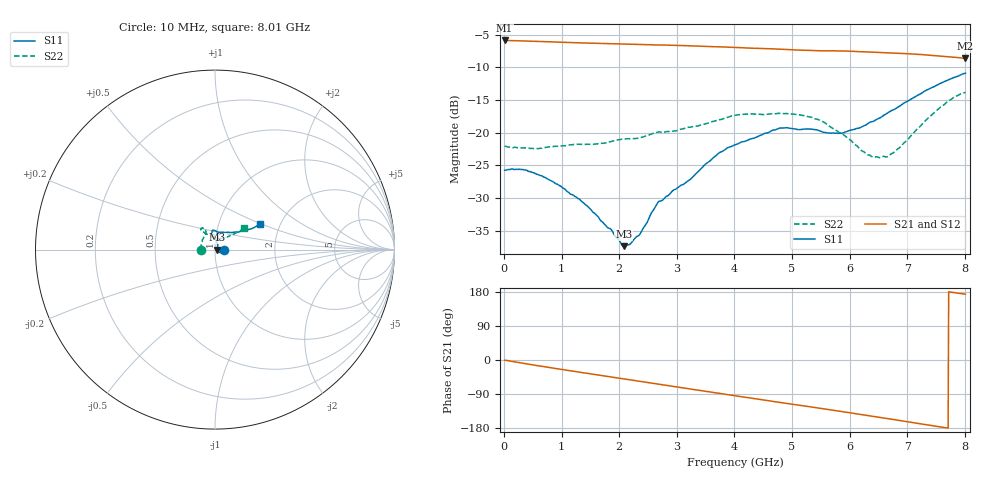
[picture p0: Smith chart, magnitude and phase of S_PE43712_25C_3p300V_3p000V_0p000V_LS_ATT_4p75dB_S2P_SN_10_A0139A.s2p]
! DEVICE ID: PE43712
! File Path: z:\PE43713\PE43713_CHAR_NOM_04292014\AMB\3p300\LS_ATT_4p75dB\PE43713_AMB_3p300V_3p000V_0p000V_LS_ATT_4p75dB_S2P_SN_10_A0139A.s2p
! Serial: 10
! Lot: A0139A
! Temp: 25C
! VDD: 3.300
! VSS: 0.000
! Control_Hi: 3.000
! Control_Lo: 0.000
! Attenuation Step: 4.75dB
! Port 1: RF1
! Port 2: RF2
! ThroughPath:1-2
! IDD: 0.0001469786
! ISS: -4.98e-008
#  Hz  S  RI  R  50
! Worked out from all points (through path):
!   801 points, 10 MHz to 8.01 GHz, reference 50 ohm
!   highest |S21| = -5.86 dB at 10 MHz (marker M1); lowest = -8.6 dB at 8.01 GHz (marker M2)
!   group delay of S21, straight-line fit = 64 ps
!   lowest |S11| = -37.4 dB at 2.08 GHz (marker M3), VSWR 1.03, Z = 51.4 + j0.00512 ohm
!   |S11| at or under -10 dB: start of sweep to end of sweep
!   |S22| runs from -23.8 to -13.8 dB; largest |S21 - S12| = 0.0015
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1e7  0.0517 -0.000115  0.5091 -0.00275  0.509 -0.00281  -0.079 0.000407
3.4e8  0.0512 -0.01  0.4982 -0.078  0.498 -0.0768  -0.0763 0.00628
6.3e8  0.0446 -0.0151  0.4803 -0.1383  0.4803 -0.1383  -0.0751 0.0123
9.6e8  0.0355 -0.0172  0.4512 -0.2009  0.4513 -0.2009  -0.0766 0.02
1.35e9  0.0255 -0.0154  0.4088 -0.2657  0.4088 -0.2658  -0.0759 0.03
1.86e9  0.0175 -0.005  0.3417 -0.3386  0.3417 -0.3385  -0.0708 0.0483
2.08e9  0.0136 4.98e-05  0.3087 -0.3656  0.3088 -0.3655  -0.0702 0.0556
2.18e9  0.0136 0.00303  0.2931 -0.3769  0.2932 -0.3767  -0.0682 0.0589
2.36e9  0.0133 0.0103  0.2632 -0.3954  0.2633 -0.3953  -0.0627 0.0668
2.68e9  0.0157 0.0252  0.2091 -0.4209  0.2092 -0.4209  -0.0531 0.0867
3.23e9  0.00737 0.0432  0.1089 -0.45  0.1089 -0.4501  -0.0518 0.0975
3.72e9  0.00178 0.0693  0.0193 -0.4546  0.0191 -0.4545  -0.0556 0.1122
4.01e9  -0.00522 0.0808  -0.0336 -0.4491  -0.0336 -0.4491  -0.0655 0.1193
4.79e9  -0.0147 0.1078  -0.1629 -0.4049  -0.163 -0.4051  -0.0791 0.1166
5.35e9  -0.00189 0.1063  -0.2405 -0.3525  -0.2404 -0.3522  -0.0775 0.1057
5.87e9  0.0266 0.0958  -0.3045 -0.2933  -0.3039 -0.2934  -0.0447 0.0869
6.38e9  0.0733 0.0967  -0.3513 -0.2197  -0.3508 -0.2196  -0.00278 0.066
6.68e9  0.1065 0.0966  -0.371 -0.1717  -0.3706 -0.1719  0.0266 0.0611
6.88e9  0.1281 0.0978  -0.381 -0.139  -0.3806 -0.139  0.0453 0.063
7.56e9  0.2059 0.1178  -0.3858 -0.0246  -0.3855 -0.0248  0.1219 0.0957
7.81e9  0.2306 0.1307  -0.3788 0.0135  -0.3786 0.0132  0.1497 0.1121
8.01e9  0.2499 0.14  -0.3697 0.041  -0.3691 0.0404  0.1638 0.1212
